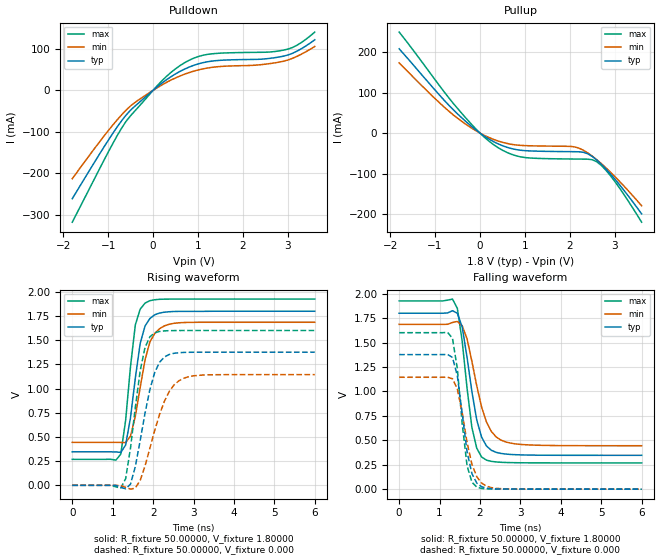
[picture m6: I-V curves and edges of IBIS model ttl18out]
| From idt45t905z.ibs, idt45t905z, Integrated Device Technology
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|   Model ttl18out
[Model]   ttl18out
Model_type   Output
Polarity   Non-Inverting
Vmeas =  0.90000V
C_comp   5.00000pF   5.00000pF   5.00000pF
[Temperature Range]   45.00000   0.14000k   -30.00000
[Voltage Range]   1.80000V   1.65000V   1.95000V
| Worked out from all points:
|   slope of the pulldown table from 0 to 0.27 V, typ, clamps not added: 11.6 ohm
|   slope of the pullup table from 0 to 0.27 V, typ, clamps not added: 14.1 ohm
|   rising waveform, R_fixture 50.00000, V_fixture 1.80000: 20-80 % time 294ps typ, 343ps min, 246ps max; typ from 0.346 V to 1.8 V
|   rising waveform, R_fixture 50.00000, V_fixture 0.000: 20-80 % time 399ps typ, 516ps min, 312ps max; typ from 0 V to 1.38 V
|   falling waveform, R_fixture 50.00000, V_fixture 1.80000: 20-80 % time 351ps typ, 424ps min, 286ps max; typ from 1.8 V to 0.346 V
|   falling waveform, R_fixture 50.00000, V_fixture 0.000: 20-80 % time 280ps typ, 331ps min, 237ps max; typ from 1.38 V to 0 V
[Pulldown]
| voltage   I(typ)   I(min)   I(max)
-1.8V     -261.1mA   -213mA     -317.7mA
-1V       -120.6mA   -97.41mA   -149mA
-600mV    -59.39mA   -47.53mA   -74.48mA
-400mV    -37.65mA   -28.88mA   -48.96mA
100mV     9.159mA    6.841mA    12.13mA
500mV     39.61mA    29.9mA     51.91mA
900mV     60mA       46.01mA    77.22mA
1.2V      68.62mA    53.53mA    86.39mA
2.5V      75.79mA    63.01mA    91.78mA
3V        85.05mA    72.93mA    99.21mA
3.3V      100.1mA    86.93mA    115mA
3.6V      121.7mA    105.6mA    140.3mA
[Pullup]
| voltage   I(typ)   I(min)   I(max)
-1.8V     208.2mA    173.4mA    249.5mA
-600mV    58.25mA    45.5mA     74.13mA
-100mV    8.512mA    6.375mA    11.27mA
200mV     -14.77mA   -10.9mA    -19.84mA
500mV     -31.12mA   -22.77mA   -42.22mA
900mV     -42.33mA   -30.33mA   -58.64mA
2.1V      -45.95mA   -33.9mA    -64.09mA
2.4V      -51.05mA   -48.94mA   -64.5mA
2.6V      -66.39mA   -65.62mA   -70.76mA
2.8V      -87.93mA   -85.25mA   -91.14mA
3V        -113.1mA   -106.9mA   -119mA
3.6V      -199.5mA   -179.5mA   -220.1mA
[Ramp]
| variable   typ   min   max
dV/dt_r   0.82620/0.39679n   0.68700/0.51975n   0.96060/0.30242n
dV/dt_f   0.87228/0.34102n   0.74826/0.41513n   0.99396/0.28281n
R_load = 50.00000
[Rising Waveform]
R_fixture = 50.00000
V_fixture = 1.80000
C_fixture = 0.000F
R_dut = 2.40000m
L_dut = 0.90000nH
C_dut = 60.00000fF
| time   V(typ)   V(min)   V(max)
0s        346.2mV    444.4mV    268.7mV
1.2ns     339.8mV    443.1mV    322.1mV
1.32ns    416.3mV    441.4mV    670.4mV
1.44ns    697.9mV    508.4mV    1.226V
1.56ns    1.108V     713.4mV    1.659V
1.68ns    1.466V     1.011V     1.821V
1.8ns     1.647V     1.296V     1.884V
2.04ns    1.764V     1.57V      1.919V
2.4ns     1.795V     1.666V     1.925V
6ns       1.8V       1.686V     1.926V
[Rising Waveform]
R_fixture = 50.00000
V_fixture = 0.000
C_fixture = 0.000F
R_dut = 2.40000m
L_dut = 0.90000nH
C_dut = 60.00000fF
| time   V(typ)   V(min)   V(max)
0s        0V         0V         0V
1.2ns     -20.59mV   -1.436mV   -29.36mV
1.32ns    -36.35mV   -21.14mV   67.99mV
1.44ns    11.94mV    -39.77mV   382.5mV
1.68ns    461.2mV    50.46mV    1.183V
1.8ns     745.8mV    199.3mV    1.425V
2.04ns    1.167V     567.6mV    1.577V
2.4ns     1.353V     970.6mV    1.599V
2.76ns    1.375V     1.107V     1.601V
6ns       1.377V     1.145V     1.601V
[Falling Waveform]
R_fixture = 50.00000
V_fixture = 1.80000
C_fixture = 0.000F
R_dut = 2.40000m
L_dut = 0.90000nH
C_dut = 60.00000fF
| time   V(typ)   V(min)   V(max)
0s        1.8V       1.686V     1.926V
1.32ns    1.826V     1.706V     1.945V
1.44ns    1.8V       1.716V     1.85V
1.56ns    1.658V     1.672V     1.514V
1.68ns    1.349V     1.539V     1.033V
1.8ns     997.9mV    1.308V     630.7mV
2.04ns    532.6mV    840.6mV    329.5mV
2.28ns    398.1mV    591.6mV    284.4mV
2.64ns    359.2mV    482.6mV    273mV
6ns       346.2mV    444.5mV    268.7mV
[Falling Waveform]
R_fixture = 50.00000
V_fixture = 0.000
C_fixture = 0.000F
R_dut = 2.40000m
L_dut = 0.90000nH
C_dut = 60.00000fF
| time   V(typ)   V(min)   V(max)
0s        1.377V     1.145V     1.601V
1.2ns     1.378V     1.145V     1.604V
1.32ns    1.347V     1.13V      1.542V
1.44ns    1.16V      1.025V     1.232V
1.56ns    775.1mV    783.2mV    670.3mV
1.68ns    384.1mV    480.3mV    240.2mV
1.8ns     159.7mV    255.5mV    71.68mV
1.92ns    62.55mV    129.1mV    22.05mV
2.4ns     2.955mV    8.545mV    1.172mV
6ns       560.9nV    2.393uV    0V
